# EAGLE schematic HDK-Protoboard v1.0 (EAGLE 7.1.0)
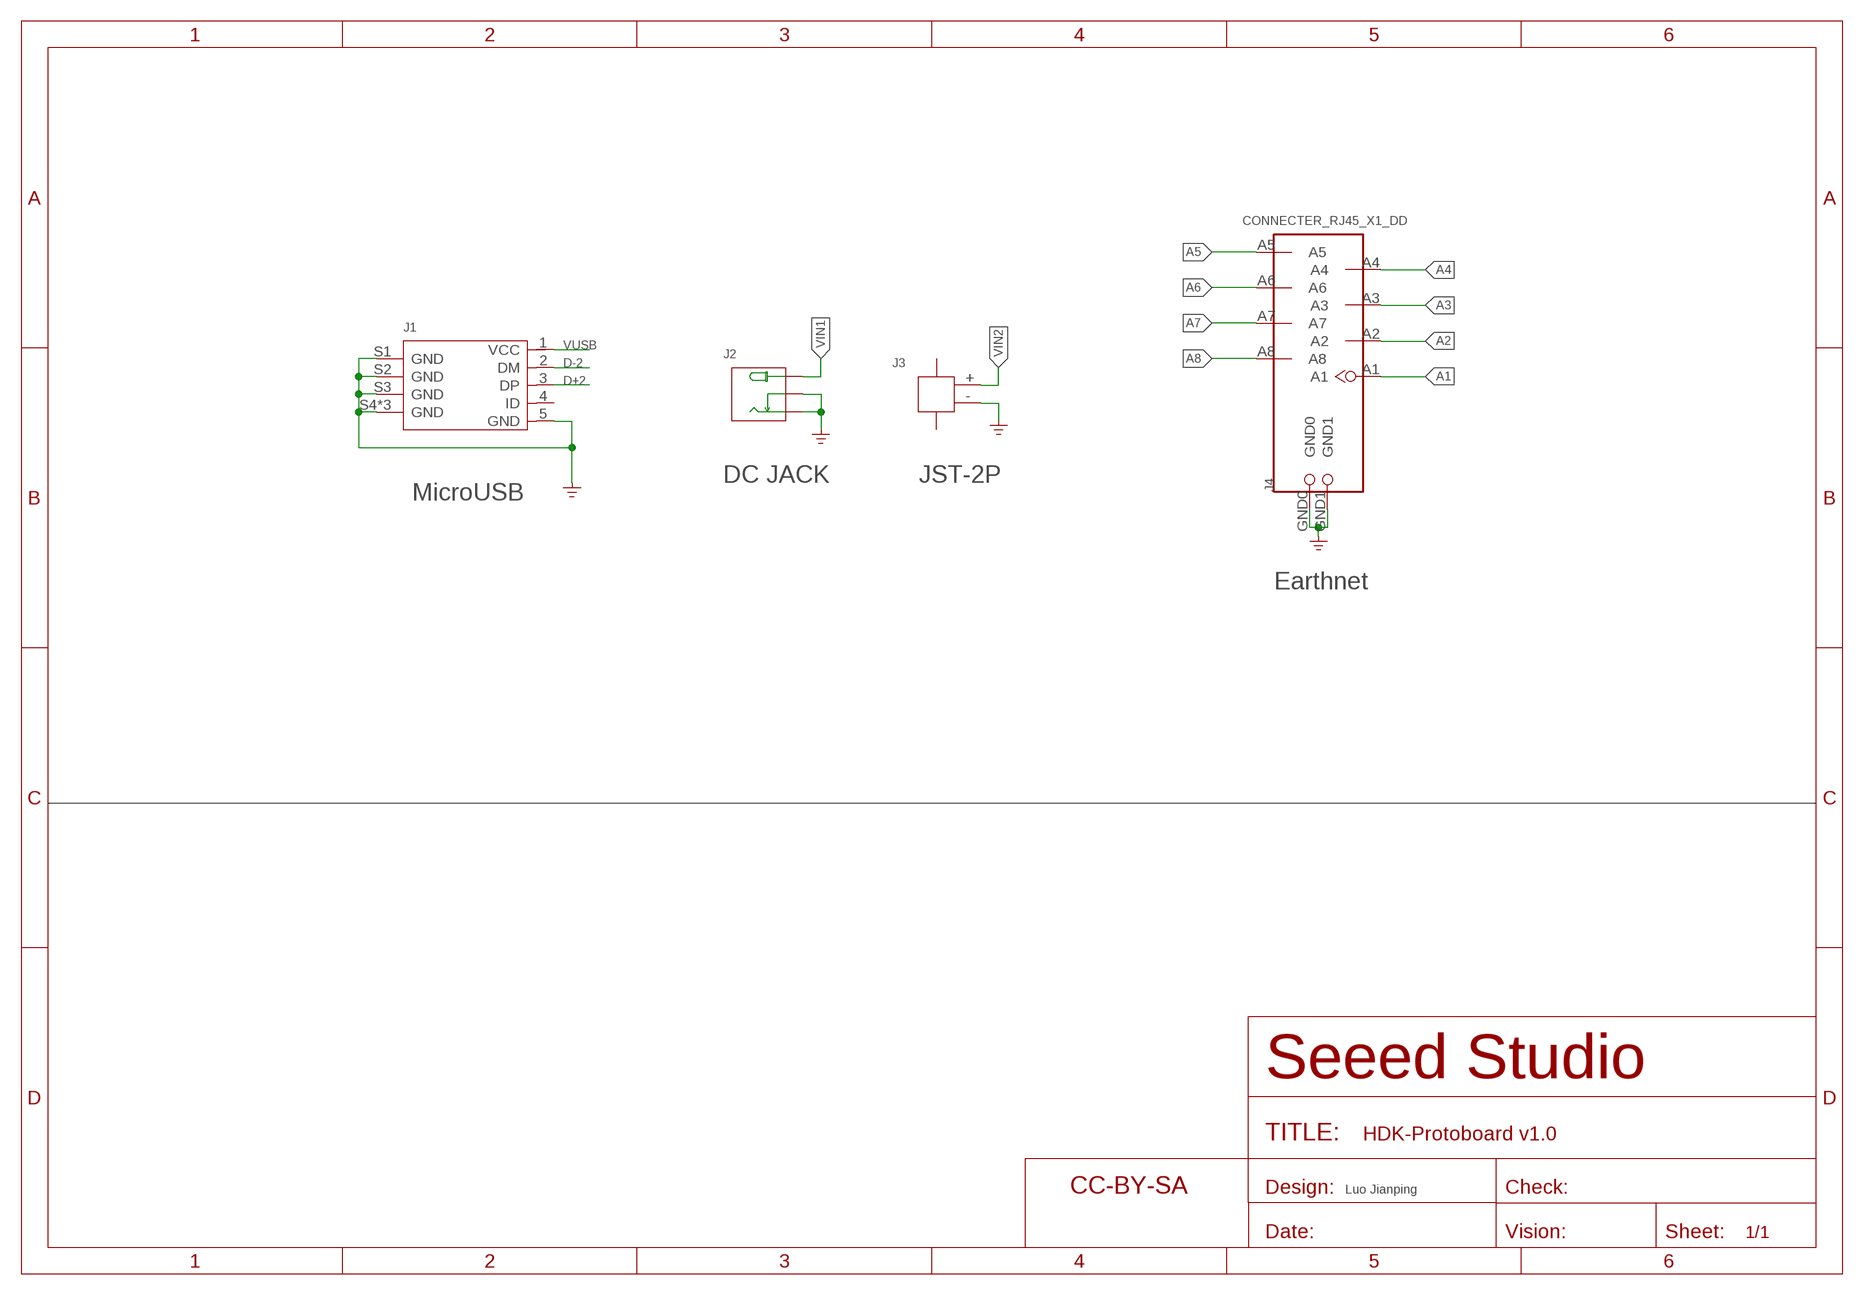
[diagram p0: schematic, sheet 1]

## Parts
FR1  SEEEDSTUDIO-OPEN-SCH-FRAME  [SEEEDSTUDIO-PCB-FRAME]
J1  MICRO-USB5+4P  [MICRO-USB5+4P-SMD-0.65-B-NO-HOLE]
J2  POWER-JACK-DC'DC-044'  [DCJ3P-11.6X9.6X7.0MM]
J3  JST-2P-SMD'2.0'  [HW2-SMD-2.0-90D]
J4  CONNECTER_RJ45_X1_DD  [RJ45-8P-20.4X16MM]

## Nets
A1: J4.A1
A2: J4.A2
A3: J4.A3
A4: J4.A4
A5: J4.A5
A6: J4.A6
A7: J4.A7
A8: J4.A8
D+2: J1.3(DP)
D-2: J1.2(DM)
GND [none1]: J1.5(GND) J1.S1(GND) J1.S2(GND) J1.S3(GND) J1.S4(GND) J1.S5(GND) J1.S6(GND) J2.- J2.CDN J3.- J4.GND0 J4.GND1 ; supply symbol labelled GND_POWER
VIN1: J2.+
VIN2: J3.+
VUSB: J1.1(VCC)
Unconnected: J1.4(ID) J3.3 J3.4

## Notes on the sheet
- DC JACK | JST-2P
- MicroUSB
- Earthnet
- Luo Jianping

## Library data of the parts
FR1 = moudle-new:SEEEDSTUDIO-OPEN-SCH-FRAME
J1 = Connector-new:MICRO-USB5+4P: 5+4P-SMD-0.65-B:320010000;5+2P-SMD-0.65-AB:340032001
J2 = Connector-new:POWER-JACK-DC: 3P-L11.6*W9.6*H7.0MM:320120002;3P-L14.2*W11.0*H9.0MM:320120003
J3 = Connector-new:JST-2P-SMD: 2P-SMD-1.0-90D:320110054;2P-SMD-2.0-90D:320110026
J4 = template:CONNECTER_RJ45_X1

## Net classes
2 gnd: width 0.305 mm, drill 0.559 mm, clearance 0.254 mm
3 none3: width 0.203 mm, drill 0.305 mm, clearance 0.203 mm
4 aref: width 0.406 mm, drill 0.61 mm, clearance 0.254 mm

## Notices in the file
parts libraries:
moudle-new: This work is licensed under the Creative Commons Attribution 4.0 International License.
To view a copy of this license,visit:
http://creativecommons.org/licenses/by-sa/4.0
moudle-new: CC-BY-SA
